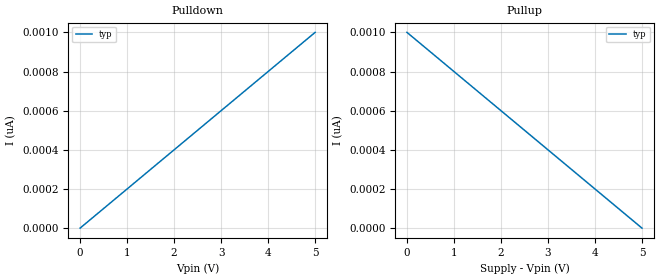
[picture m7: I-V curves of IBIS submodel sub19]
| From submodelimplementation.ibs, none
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| ... Off_delay is not valid with both pullup and pulldown specified
[Submodel] sub19
Submodel_type Bus_hold
[Submodel Spec]
V_trigger_r   1.2   1   1.6
V_trigger_f   3.6   3.8   2.9
Off_delay   2n   1n   3n
[Pulldown]
0V        0A         NA         NA
5V        1nA        NA         NA
[Pullup]
0V        1nA        NA         NA
5V        0A         NA         NA
[Ramp]
dV/dt_r		1/1n   NA   NA
dV/dt_f		1/1n   NA   NA
